| TEXAS INSTRUMENTS INCORPORATED
| Standard Linear and Logic Group
| IBIS Model of SN74AVC16827
| 20-BitBuffer/Driver With 3-State Outputs
| This file contains package information for the following:
|  TSSOP 56-pin (DGG) package as [Component] AVC16827_DGG
|  TVSOP 56-pin (DGV) package as [Component] AVC16827_DGV
| This device can be powered at the following Vccs:
|  3.3 volt Vcc
|  2.5 volt Vcc
|  1.8 volt Vcc
|  1.5 volt Vcc
|  1.2 volt Vcc
| This file provides unique models under the [Model Selector] for each Vcc.
| For operation at a specific Vcc, select the appropriate model after each
| [Model Selector] keyword.
[IBIS Ver]   3.2
[Comment char]  |_char
[File Name]   sn74avc16827.ibs
[File Rev]   1.1 | a_die
[Date]   February 20, 2004
[Source]   Data created from TI-SPICE simulations at TI-SLL.
[Notes]   The following is an IBIS list for the AVC16827.
   Please contact sllibis@ti.com with questions and
   comments concerning SLL IBIS models.
   - FILE REV HISTORY
   - 1.1 Release IBIS file on 02/20/04
   - Power-clamp data has been deleted since there is no
   power-clamp diode in the device.
   - IBIS 3.2 SYNTAX CANNOT DESCRIBE THE CHARACTERISTICS OF
   ANY OUTPUT STRUCTURES THAT DYNAMICALLY CHANGES THE
   IMPEDANCES DURING THE TRANSITION. THIS DEVICE USE SIMILAR
   OUTPUT STRUCTURE AND THEREFORE THE SIMULATION RESULTS
   MAY NOT BE ACCURATE. TI RECOMMENDS THE USE OF SPICE
   SIMULATION WHEN SIMULATION ACCURACY IS IMPORTANT.
[Disclaimer] Property of Texas Instruments Incorporated.  Unauthorized
   reproduction and/or distribution is strictly prohibited.
   This product is protected under copyright law.
   Created  2003, (C) Copyright  2003, Texas Instruments
   Incorporated, All Rights Reserved
   UNLESS THERE IS A SIGNED, WRITTEN AGREEMENT TO THE
   CONTRARY, TEXAS INSTRUMENTS (TI) IS PROVIDING THE IBIS
   MODELS  AND WITHOUT ANY WARRANTY, EXPRESSED OR
   IMPLIED.  TI assumes no liability for:
   1) the accuracy of the IBIS models provided to your
   company;
   2) the proper functioning of these IBIS Models in your
   design or for any resulting applications; or
   3) infringement of patents, copyrights or intellectual
   property rights resulting from your use of these IBIS
   models.
   TI provides IBIS Models as a service to our customers.
   You and your company shall not distribute, sell or give
   these models to anyone else without prior written
   permission from TI.
   TI reserves the right to make changes to our products or
   to discontinue any semiconductor product or service
   without notice, and advises our customers to obtain the
   latest version of relevant information to verify, before
   placing orders, that the information being relied on is
   current.
   Please be aware that your receipt and use of the IBIS
   information provided shall serve as acceptance of these
   terms and conditions.  If you do not accept these terms,
   you should return or destroy the IBIS models and any
   other accompanying information immediately.
| Component AVC16827_DGG 56-pin TSSOP
[Component]   AVC16827_DGG
[Manufacturer]   Texas Instruments, Inc.
[Package]
|   typ   min   max
R_pkg   4.500e-02   3.500e-02   6.200e-02
L_pkg   3.324e-09   2.403e-09   5.094e-09
C_pkg   5.640e-13   3.410e-13   9.140e-13
[Pin]   signal_name   model_name   R_pin   L_pin   C_pin
1   1OE1   AVC16827_NOE   6.200e-02   5.094e-09   8.560e-13
2   1Y1   AVC16827_OUT   6.100e-02   4.621e-09   9.020e-13
3   1Y2   AVC16827_OUT   6.000e-02   4.316e-09   8.020e-13
4   GND   GND   5.900e-02   3.968e-09   6.980e-13
5   1Y3   AVC16827_OUT   5.700e-02   3.716e-09   6.490e-13
6   1Y4   AVC16827_OUT   4.200e-02   3.517e-09   6.530e-13
7   VCC   POWER   4.100e-02   3.160e-09   5.700e-13
8   1Y5   AVC16827_OUT   3.900e-02   2.981e-09   4.820e-13
9   1Y6   AVC16827_OUT   3.900e-02   2.808e-09   4.470e-13
10   1Y7   AVC16827_OUT   3.800e-02   2.715e-09   4.090e-13
11   GND   GND   4.100e-02   2.675e-09   3.910e-13
12   1Y8   AVC16827_OUT   3.900e-02   2.536e-09   3.660e-13
13   1Y9   AVC16827_OUT   3.900e-02   2.457e-09   3.480e-13
14   1Y10   AVC16827_OUT   3.800e-02   2.411e-09   3.530e-13
15   2Y1   AVC16827_OUT   3.900e-02   2.456e-09   3.550e-13
16   2Y2   AVC16827_OUT   3.900e-02   2.471e-09   3.490e-13
17   2Y3   AVC16827_OUT   4.000e-02   2.580e-09   3.700e-13
18   GND   GND   3.800e-02   2.651e-09   3.890e-13
19   2Y4   AVC16827_OUT   3.800e-02   2.739e-09   4.110e-13
20   2Y5   AVC16827_OUT   3.900e-02   2.838e-09   4.490e-13
21   2Y6   AVC16827_OUT   3.800e-02   2.988e-09   4.840e-13
22   VCC   POWER   3.800e-02   3.104e-09   5.640e-13
23   2Y7   AVC16827_OUT   4.000e-02   3.427e-09   6.380e-13
24   2Y8   AVC16827_OUT   5.600e-02   3.654e-09   6.410e-13
25   GND   GND   5.700e-02   3.932e-09   7.000e-13
26   2Y9   AVC16827_OUT   5.800e-02   4.257e-09   8.060e-13
27   2Y10   AVC16827_OUT   5.700e-02   4.580e-09   9.140e-13
28   2OE1   AVC16827_NOE   5.900e-02   5.038e-09   8.610e-13
29   2OE2   AVC16827_NOE   6.000e-02   5.058e-09   8.580e-13
30   2A10   AVC16827_IN   5.600e-02   4.543e-09   9.040e-13
31   2A9   AVC16827_IN   5.700e-02   4.241e-09   8.020e-13
32   GND   GND   5.900e-02   3.933e-09   6.990e-13
33   2A8   AVC16827_IN   5.600e-02   3.616e-09   6.370e-13
34   2A7   AVC16827_IN   3.700e-02   3.368e-09   6.400e-13
35   VCC   POWER   3.600e-02   3.024e-09   5.630e-13
36   2A6   AVC16827_IN   3.500e-02   2.876e-09   4.740e-13
37   2A5   AVC16827_IN   3.500e-02   2.745e-09   4.440e-13
38   2A4   AVC16827_IN   3.700e-02   2.683e-09   4.050e-13
39   GND   GND   3.800e-02   2.603e-09   3.820e-13
40   2A3   AVC16827_IN   3.800e-02   2.510e-09   3.620e-13
41   2A2   AVC16827_IN   3.600e-02   2.412e-09   3.410e-13
42   2A1   AVC16827_IN   3.800e-02   2.416e-09   3.490e-13
43   1A10   AVC16827_IN   3.800e-02   2.403e-09   3.490e-13
44   1A9   AVC16827_IN   3.700e-02   2.429e-09   3.410e-13
45   1A8   AVC16827_IN   3.600e-02   2.483e-09   3.580e-13
46   GND   GND   3.700e-02   2.614e-09   3.810e-13
47   1A7   AVC16827_IN   3.500e-02   2.669e-09   4.020e-13
48   1A6   AVC16827_IN   3.600e-02   2.763e-09   4.420e-13
49   1A5   AVC16827_IN   3.600e-02   2.942e-09   4.780e-13
50   VCC   POWER   3.500e-02   3.053e-09   5.640e-13
51   1A4   AVC16827_IN   3.600e-02   3.408e-09   6.410e-13
52   1A3   AVC16827_IN   5.800e-02   3.698e-09   6.410e-13
53   GND   GND   5.900e-02   3.974e-09   6.970e-13
54   1A2   AVC16827_IN   6.100e-02   4.327e-09   8.020e-13
55   1A1   AVC16827_IN   6.100e-02   4.624e-09   9.050e-13
56   1OE2   AVC16827_NOE   6.000e-02   5.063e-09   8.580e-13
| Component AVC16827_DGV 56-pin TVSOP
[Component]   AVC16827_DGV
[Manufacturer]   Texas Instruments, Inc.
[Package]
|   typ   min   max
R_pkg   6.300e-02   5.000e-02   8.400e-02
L_pkg   2.945e-09   2.394e-09   3.939e-09
C_pkg   3.910e-13   2.710e-13   5.880e-13
[Pin]   signal_name   model_name   R_pin   L_pin   C_pin
1   1OE1   AVC16827_NOE   6.800e-02   3.933e-09   5.880e-13
2   1Y1   AVC16827_OUT   6.800e-02   3.568e-09   5.870e-13
3   1Y2   AVC16827_OUT   7.600e-02   3.464e-09   5.150e-13
4   GND   GND   8.400e-02   3.444e-09   4.590e-13
5   1Y3   AVC16827_OUT   8.100e-02   3.277e-09   4.270e-13
6   1Y4   AVC16827_OUT   7.400e-02   3.136e-09   3.870e-13
7   VCC   POWER   6.900e-02   2.970e-09   4.010e-13
8   1Y5   AVC16827_OUT   5.000e-02   2.785e-09   3.790e-13
9   1Y6   AVC16827_OUT   5.100e-02   2.685e-09   3.200e-13
10   1Y7   AVC16827_OUT   5.300e-02   2.611e-09   3.160e-13
11   GND   GND   5.300e-02   2.495e-09   2.970e-13
12   1Y8   AVC16827_OUT   5.300e-02   2.435e-09   2.920e-13
13   1Y9   AVC16827_OUT   5.500e-02   2.412e-09   2.850e-13
14   1Y10   AVC16827_OUT   5.600e-02   2.401e-09   2.730e-13
15   2Y1   AVC16827_OUT   5.500e-02   2.401e-09   2.730e-13
16   2Y2   AVC16827_OUT   5.500e-02   2.399e-09   2.840e-13
17   2Y3   AVC16827_OUT   5.400e-02   2.406e-09   2.890e-13
18   GND   GND   5.300e-02   2.450e-09   2.930e-13
19   2Y4   AVC16827_OUT   5.100e-02   2.544e-09   3.110e-13
20   2Y5   AVC16827_OUT   5.100e-02   2.626e-09   3.150e-13
21   2Y6   AVC16827_OUT   5.000e-02   2.727e-09   3.690e-13
22   VCC   POWER   6.500e-02   2.903e-09   3.930e-13
23   2Y7   AVC16827_OUT   7.500e-02   3.091e-09   3.860e-13
24   2Y8   AVC16827_OUT   8.200e-02   3.272e-09   4.280e-13
25   GND   GND   8.200e-02   3.393e-09   4.570e-13
26   2Y9   AVC16827_OUT   7.300e-02   3.380e-09   5.080e-13
27   2Y10   AVC16827_OUT   7.100e-02   3.577e-09   5.800e-13
28   2OE1   AVC16827_NOE   6.800e-02   3.937e-09   5.740e-13
29   2OE2   AVC16827_NOE   6.900e-02   3.923e-09   5.690e-13
30   2A10   AVC16827_IN   6.400e-02   3.536e-09   5.740e-13
31   2A9   AVC16827_IN   7.600e-02   3.428e-09   5.170e-13
32   GND   GND   8.100e-02   3.395e-09   4.680e-13
33   2A8   AVC16827_IN   8.000e-02   3.255e-09   4.310e-13
34   2A7   AVC16827_IN   7.100e-02   3.064e-09   3.860e-13
35   VCC   POWER   6.100e-02   2.878e-09   3.890e-13
36   2A6   AVC16827_IN   5.000e-02   2.710e-09   3.630e-13
37   2A5   AVC16827_IN   5.000e-02   2.606e-09   3.110e-13
38   2A4   AVC16827_IN   5.200e-02   2.534e-09   3.060e-13
39   GND   GND   5.200e-02   2.439e-09   2.890e-13
40   2A3   AVC16827_IN   5.300e-02   2.399e-09   2.860e-13
41   2A2   AVC16827_IN   5.500e-02   2.394e-09   2.820e-13
42   2A1   AVC16827_IN   5.500e-02   2.398e-09   2.710e-13
43   1A10   AVC16827_IN   5.600e-02   2.396e-09   2.710e-13
44   1A9   AVC16827_IN   5.400e-02   2.402e-09   2.830e-13
45   1A8   AVC16827_IN   5.400e-02   2.423e-09   2.880e-13
46   GND   GND   5.300e-02   2.474e-09   2.920e-13
47   1A7   AVC16827_IN   5.100e-02   2.569e-09   3.090e-13
48   1A6   AVC16827_IN   5.100e-02   2.638e-09   3.130e-13
49   1A5   AVC16827_IN   5.100e-02   2.742e-09   3.660e-13
50   VCC   POWER   6.400e-02   2.917e-09   3.900e-13
51   1A4   AVC16827_IN   7.400e-02   3.083e-09   3.830e-13
52   1A3   AVC16827_IN   8.100e-02   3.249e-09   4.300e-13
53   GND   GND   8.300e-02   3.400e-09   4.550e-13
54   1A2   AVC16827_IN   7.500e-02   3.427e-09   5.050e-13
55   1A1   AVC16827_IN   7.100e-02   3.585e-09   5.780e-13
56   1OE2   AVC16827_NOE   6.900e-02   3.939e-09   5.810e-13
| Model AVC16827_IN
[Model Selector]   AVC16827_IN
AVC16827_IN_33   3.3 volt Vcc
AVC16827_IN_25   2.5 volt Vcc
AVC16827_IN_18   1.8 volt Vcc
AVC16827_IN_15   1.5 volt Vcc
AVC16827_IN_12   1.2 volt Vcc
| Model AVC16827_NOE
[Model Selector]   AVC16827_NOE
AVC16827_NOE_33   3.3 volt Vcc
AVC16827_NOE_25   2.5 volt Vcc
AVC16827_NOE_18   1.8 volt Vcc
AVC16827_NOE_15   1.5 volt Vcc
AVC16827_NOE_12   1.2 volt Vcc
| Model AVC16827_OUT
[Model Selector]   AVC16827_OUT
AVC16827_OUT_33   3.3 volt Vcc
AVC16827_OUT_25   2.5 volt Vcc
AVC16827_OUT_18   1.8 volt Vcc
AVC16827_OUT_15   1.5 volt Vcc
AVC16827_OUT_12   1.2 volt Vcc
| Models and submodels in the file (15): AVC16827_IN_33 (Input), AVC16827_IN_25 (Input), AVC16827_IN_18 (Input), AVC16827_IN_15 (Input), AVC16827_IN_12 (Input), AVC16827_NOE_33 (Input), AVC16827_NOE_25 (Input), AVC16827_NOE_18 (Input), AVC16827_NOE_15 (Input), AVC16827_NOE_12 (Input), AVC16827_OUT_33 (3-state), AVC16827_OUT_25 (3-state), AVC16827_OUT_18 (3-state), AVC16827_OUT_15 (3-state), AVC16827_OUT_12 (3-state)
